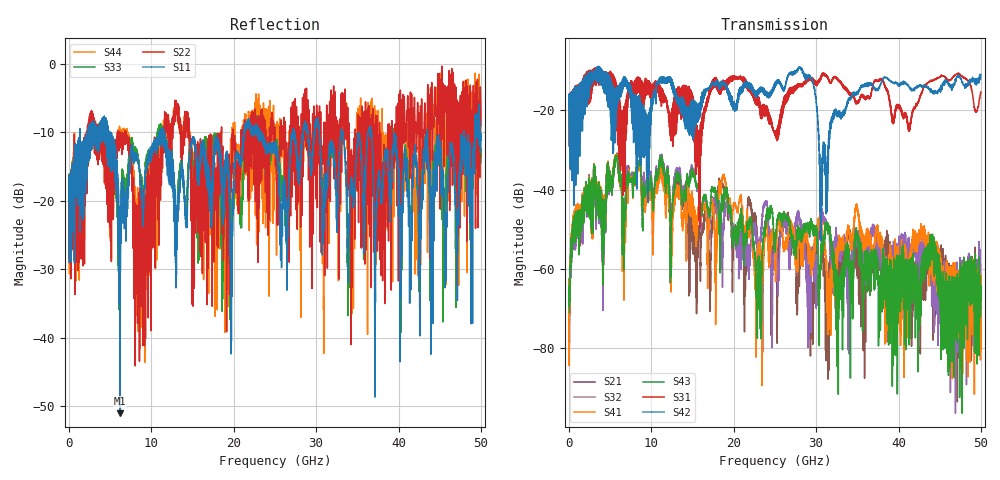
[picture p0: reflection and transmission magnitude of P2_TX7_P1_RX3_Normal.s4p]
!Keysight Technologies,N5225B,MY57041031,A.13.20.10
!Date: Friday, May 31, 2019 11:18:33
!Correction: S11(Full 4 Port(1,2,3,4))
!S12(Full 4 Port(1,2,3,4))
!S13(Full 4 Port(1,2,3,4))
!S14(Full 4 Port(1,2,3,4))
!S21(Full 4 Port(1,2,3,4))
!S22(Full 4 Port(1,2,3,4))
!S23(Full 4 Port(1,2,3,4))
!S24(Full 4 Port(1,2,3,4))
!S31(Full 4 Port(1,2,3,4))
!S32(Full 4 Port(1,2,3,4))
!S33(Full 4 Port(1,2,3,4))
!S34(Full 4 Port(1,2,3,4))
!S41(Full 4 Port(1,2,3,4))
!S42(Full 4 Port(1,2,3,4))
!S43(Full 4 Port(1,2,3,4))
!S44(Full 4 Port(1,2,3,4))
!S4P File: Measurements: <S11,S12,S13,S14>,
!<S21,S22,S23,S24>,
!<S31,S32,S33,S34>,
!<S41,S42,S43,S44>:
# Hz S  dB  R 50.0
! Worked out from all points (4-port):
!   5000 points, 10 MHz to 50 GHz, reference 50 ohm
!   strongest paths, dB at 10 MHz, 12.51 GHz, 25.01 GHz, 37.51 GHz, 50 GHz:
!     S42: -19.7, -14.3, -13.4, -14.9, -11.0
!     S31: -19.6, -21.1, -25.9, -12.8, -15.4
!     S43: -70.9, -45.3, -55.2, -62.0, -71.9
!     S41: -71.9, -51.2, -55.0, -52.1, -67.0
!     S32: -64.3, -43.6, -54.8, -57.1, -64.7
!     S21: -64.1, -46.7, -52.9, -55.1, -62.2
!   lowest |S11| = -51.1 dB at 6.18 GHz (marker M1), VSWR 1.01, Z = 50.1 - j0.263 ohm
!   |S11| at or under -10 dB: 4.96 GHz to 11.03 GHz (6.066 GHz wide, 75.9 % of centre); 11.57 GHz to 21.26 GHz (9.684 GHz wide, 59 % of centre); 36.74 GHz to 43.5 GHz (6.761 GHz wide, 16.9 % of centre)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
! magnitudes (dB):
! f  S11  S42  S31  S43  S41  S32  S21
! 10 MHz  -20.1  -19.7  -19.6  -70.9  -71.9  -64.3  -64.1
! 6.18 GHz  -51.1  -13.9  -18.2  -36.6  -36.9  -36.4  -36.2
! 28.07 GHz  -13.7  -9.2  -13.8  -52.2  -52.0  -47.9  -54.5
! 29.14 GHz  -11.7  -11.5  -12.1  -49.5  -56.7  -64.9  -68.9
! 30.63 GHz  -17.0  -40.7  -11.4  -54.5  -48.2  -45.5  -51.8
! 31.54 GHz  -14.9  -28.6  -12.7  -49.4  -71.5  -50.9  -72.6
! 50 GHz  -11.1  -11.0  -15.4  -71.9  -67.0  -64.7  -62.2
